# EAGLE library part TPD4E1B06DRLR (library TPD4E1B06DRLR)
Bidirectional Quad-Channel High-Speed ESD Protection Device Source: Datasheet
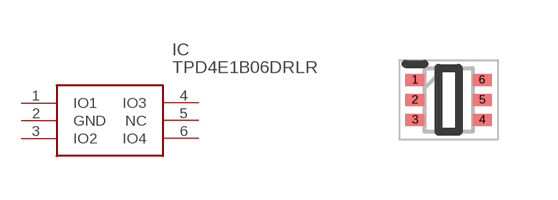
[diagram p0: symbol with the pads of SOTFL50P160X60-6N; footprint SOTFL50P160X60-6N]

Designator prefix IC

## TPD4E1B06DRLR (Description: Bidirectional Quad-Channel High-Speed ESD Protection Device; Height: 0.6mm; Manufacturer_Name: Texas Instruments; Manufacturer_Part_Number: TPD4E1B06DRLR; Mouser_Part_Number: 595-TPD4E1B06DRLR; Mouser_Price-Stock: https://www.mouser.co.uk/ProductDetail/Texas-Instruments/TPD4E1B06DRLR?qs=1MXlzafEN387aRSX0e2MEQ%3D%3D)  [SOTFL50P160X60-6N]
1  IO1
2  GND
3  IO2
4  IO3
5  NC  nc
6  IO4

## Footprint SOTFL50P160X60-6N (pad centres in mm)
DRL0006A
smd 0.475 x 0.3: 1 -0.838,0.5; 2 -0.838,0; 3 -0.838,-0.5; 4 0.838,-0.5; 5 0.838,0; 6 0.838,0.5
